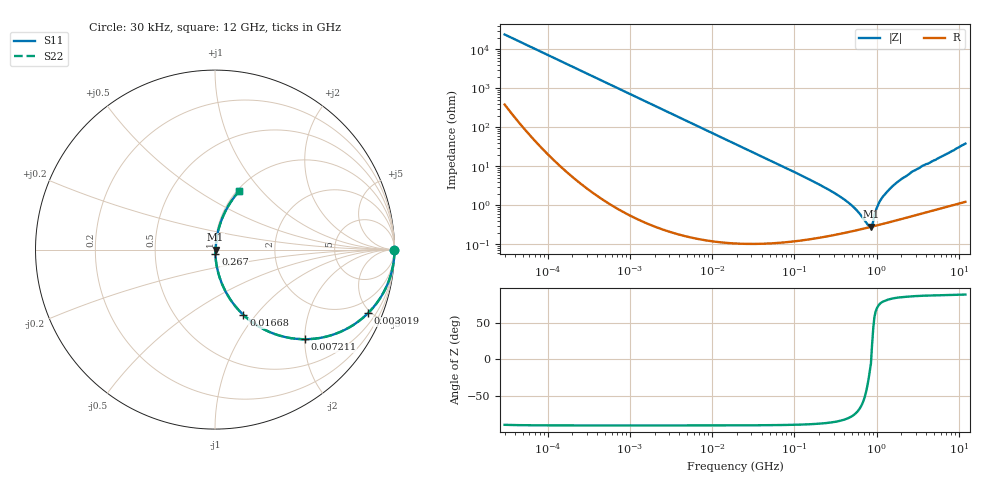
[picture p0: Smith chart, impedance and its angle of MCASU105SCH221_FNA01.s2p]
! MCASU105SCH221_FNA01  S-PARAMETER MODEL  ( General Type )
! Model Generated by TAIYO YUDEN Corporation (http://www.ty-top.com)
! Version 1.0
! TAIYO YUDEN Control No. 130207
! Copyright(c) 2013 TAIYO YUDEN CO.,LTD. All Rights Reserved.
! Product Description (link to TY-COMPAS)
! https://ds.yuden.co.jp/TYCOMPAS/or/detail?pn=MCASU105SCH221JFNA01&u=M
! Products Name : Multilayer Ceramic Capacitors
! Characteristics :
!  Capacitance : 220 pF , Rated Voltage : 50V , TCC : CH / C0H
!  Case Size : 1.0 x 0.5 / 0.039 x 0.02 [mm/inch] , Thickness : 0.5 / 0.02 [mm/inch]
!  (Conditions: Temperature = 25 degC , DC Bias Current/Voltage = 0A / 0V)
! External Node Assignments :
!  1  o---| |---o  2
! GND o---------o GND
! Frequency Range : 30000Hz  -  12GHz  [ 401 STEP ]
# MHz S RI R 50
! Freq[MHz].  S11 Real  S11 Imag  S21 Real  S21 Imag  S12 Real  S12 Imag  S22 Real  S22 Imag
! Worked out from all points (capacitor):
!   401 points, 30 kHz to 12 GHz, reference 50 ohm
!   read as one part in series: C = 220 pF near 32 kHz
!   lowest |Z| = 281 mohm at 852.6 MHz (marker M1)
!   series resonance near 858.5 MHz, so ESL is about 160 pH
!   S11 on the Smith chart (normalised r, x): 30 kHz: open; 3.019 MHz: 1.00, -4.79; 7.211 MHz: 1.00, -2.01; 16.68 MHz: 1.00, -0.87; 267 MHz: 1.00, -0.05; 12 GHz: 1.02, +0.77
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0.03  0.9999 -0.00415  8.34e-05 0.00415  8.34e-05 0.00415  0.9999 -0.00415
0.260295  0.9987 -0.0359  0.00134 0.0359  0.00134 0.0359  0.9987 -0.0359
0.858335  0.986 -0.117  0.014 0.117  0.014 0.117  0.986 -0.117
2.258455  0.9109 -0.2844  0.0891 0.2844  0.0891 0.2844  0.9109 -0.2844
3.018962  0.8514 -0.3553  0.1486 0.3553  0.1486 0.3553  0.8514 -0.3553
7.211021  0.5014 -0.4993  0.4986 0.4993  0.4986 0.4993  0.5014 -0.4993
16.67749  0.1588 -0.3642  0.8412 0.3642  0.8412 0.3642  0.1588 -0.3642
18.97367  0.1274 -0.3321  0.8726 0.3321  0.8726 0.3321  0.1274 -0.3321
51.55976  0.0202 -0.1368  0.9798 0.1368  0.9798 0.1368  0.0202 -0.1368
164.6252  0.00316 -0.0421  0.9968 0.0421  0.9968 0.0421  0.00316 -0.0421
267.0383  0.00223 -0.0244  0.9978 0.0244  0.9978 0.0244  0.00223 -0.0244
477.1624  0.00221 -0.0105  0.9978 0.0105  0.9978 0.0105  0.00221 -0.0105
598.0015  0.00238 -0.0063  0.9976 0.0063  0.9976 0.0063  0.00238 -0.0063
774.0045  0.00266 -0.00187  0.9973 0.00187  0.9973 0.00187  0.00266 -0.00187
852.6267  0.00279 -0.000277  0.9972 0.000277  0.9972 0.000277  0.00279 -0.000277
909.4299  0.00289 0.0026  0.9971 -0.0026  0.9971 -0.0026  0.00289 0.0026
1001.808  0.0031 0.00787  0.9969 -0.00787  0.9969 -0.00787  0.0031 0.00787
1068.55  0.00326 0.011  0.9967 -0.011  0.9967 -0.011  0.00326 0.011
1428.372  0.00431 0.0252  0.9957 -0.0252  0.9957 -0.0252  0.00431 0.0252
2811.574  0.011 0.0748  0.989 -0.0748  0.989 -0.0748  0.011 0.0748
6935.754  0.0469 0.1902  0.9531 -0.1902  0.9531 -0.1902  0.0469 0.1902
12000  0.1358 0.3269  0.8642 -0.3269  0.8642 -0.3269  0.1358 0.3269
